| IBIS file 3599z.ibs created by s2ibis2 version 1.1
| North Carolina State University Electronics Research Laboratory  1995
[IBIS ver]   2.1
[File name]   70v3599bf.ibs
[File Rev]   2.0
|1.0 : Original Version - Wei-Ling Chang
|2.0 : Replaced I/O and Input models with 70V659 ADC models - Sunil Kashyap
[Source]   Integrated Device Technology, Inc.
[Notes]   1.Temperatures: typ=25C, min=100C, max=0C 2.RRmp rates based
   on 50 ohm load. 3. Both inpad and iopad have 2 models each.
   (JTAG pins have one model.)
   iopad: standard 3.3V I/O model
   inpad: standard 3.3V input pad model
   iopad25: For 2.5V I/O supply
   inpad25: For 2.5V I/O supply.
   To use 2.%V models at any port, use iopad25 and inpad25
   as the model definition in pin defie section of the IBIS
   file.  JTAG pins only have models for 3.3V I/O voltage.
[Disclaimer] Integrated Device Technology, Inc. ("IDT") hereby grants the
   user of this IBIS model a non-exclusive, nontransferable
   license to use this IBIS model under the following terms. The
   user is granted this license only to use the IBIS model and is
   not granted rights to sell, copy (except as needed to run the
   IBIS model), rent, lease or sub-license the IBIS model in
   whole or in part, or in modified form to anyone. The User may
   modify the IBIS model to suit its specific applications, but
   rights to derivative works and such modifications shall belong
   to IDT. This IBIS model is provided on an AS IS" basis and IDT
   makes absolutely no warranty with respect to the information
   contained herein. IDT DISCLAIMS AND CUSTOMER WAIVES ALL
   WARRANTIES, EXPRESS AND IMPLIED, INCLUDING WARRANTIES OF
   MERCHANTABILITY AND FITNESS FOR A PARTICULAR PURPOSE. THE
   ENTIRE RISK AS TO QUALITY AND PERFORMANCE IS WITH THE USER
   ACCORDINGLY, IN NO EVENT SHALL IDT BE LIABLE FOR ANY DIRECT OR
   INDIRECT DAMAGES, WHETHER IN CONTRACT OR TORT, INCLUDING ANY
   LOST PROFITS OR OTHER INCIDENTAL, CONSEQUENTIAL, EXEMPLARY, OR
   PUNITIVE DAMAGES ARISING OUT OF THE USE OR APPLICATION OF THE
   IBIS model. Further, IDT reserves the right to make changes
   without notice to any product herein to improve reliability,
   function, or design. IDT does not convey any license under
   patent rights or any other intellectual property rights,
   including those of third parties. IDT is not obligated to
   provide maintenance or support for the licensed IBIS model.
[Copyright]   Copyright 2004, Integrated Device Technology, Inc. all rights
   reserved
|   Component idt70v3599z
[Component]   idt70v3599z
[Manufacturer]   Integrated Device Technology
[Package]
| variable   typ   min   max
R_pkg   100.00000m   50.00000m   0.30000
L_pkg   4.00000nH   3.20000nH   5.50000nH
C_pkg   0.64000pF   0.50000pF   0.70000pF
[Pin]  signal_name   model_name   R_pin   L_pin   C_pin
A1   io19l   iopad
C2   io19r   iopad
D4   io20l   iopad
B1   io20r   iopad
C1   VDDQ   POWER
D2   GND   GND
D3   io21l   iopad
E4   io21r   iopad
D1   io22l   iopad
E2   io22r   iopad
E3   VDDQ   POWER
F4   GND   GND
E1   io23l   iopad
F2   io23r   iopad
F3   io24l   iopad
G4   io24r   iopad
F1   VDDQ   POWER
G2   GND   GND
G3   io25l   iopad
H4   io25r   iopad
G1   io26l   iopad
H2   io26r   iopad
H3   VDDQ   POWER
J4   GND   GND
H1   VDD   POWER
J2   VDD   POWER
J3   GND   GND
K4   GND   GND
J1   VDDQ   POWER
K2   GND   GND
K3   io27r   iopad
L4   io27l   iopad
K1   io28r   iopad
L2   io28l   iopad
L3   VDDQ   POWER
M4   GND   GND
L1   io29r   iopad
M2   io29l   iopad
M3   io30r   iopad
N4   io30l   iopad
M1   VDDQ   POWER
N2   GND   GND
N3   io31r   iopad
N1   io31l   iopad
P1   io32r   iopad
P2   io32l   iopad
P3   VDDQ   POWER
R1   GND   GND
T1   io33r   iopad
R2   io33l   iopad
R3   io34r   iopad
T2   io34l   iopad
U1   GND   GND
T3   VDDQ   POWER
P4   io35r   iopad
U2   io35l   iopad
U3   plftr#   inpad
P6   a16r   inpad
U5   a15r   inpad
T6   a14r   inpad
R6   a13r   inpad
P7   a12r   inpad
U6   a11r   inpad
T7   a10r   inpad
R7   a9r   inpad
P8   a8r   inpad
U7   a7r   inpad
T8   be3r#   inpad
R8   be2r#   inpad
P9   be1r#   inpad
U8   be0r#   inpad
T9   ce1r   inpad
R9   ce0r   inpad
P10   VDD   POWER
U9   VDD   POWER
T10   GND   GND
R10   GND   GND
P11   clkr   inpad
U10   oe#   inpad
T11   rwr#   inpad
R11   adsr#   inpad
P12   cntenr#   inpad
U11   repeatr#   inpad
T12   a6r   inpad
R12   a5r   inpad
P13   a4r   inpad
U12   a3r   inpad
T13   a2r   inpad
R13   a1r   inpad
U13   a0r   inpad
U14   VDD   POWER
T14   GND   GND
R14   GND   GND
U15   optr   inpad
U16   io0l   iopad
T15   io0r   iopad
R15   VDDQ   POWER
T16   GND   GND
U17   io1l   iopad
R16   io1r   iopad
P14   io2l   iopad
T17   io2r   iopad
R17   VDDQ   POWER
P16   GND   GND
P15   io3l   iopad
N14   io3r   iopad
P17   io4l   iopad
N16   io4r   iopad
N15   VDDQ   POWER
M14   GND   GND
N17   io5l   iopad
M16   io5r   iopad
M15   io6l   iopad
L14   io6r   iopad
M17   VDDQ   POWER
L16   GND   GND
L15   io7l   iopad
K14   io7r   iopad
L17   io8l   iopad
K16   io8r   iopad
K15   VDDQ   POWER
J14   GND   GND
K17   GND   GND
J16   GND   GND
J15   VDD   POWER
H14   VDD   POWER
J17   VDDQ   POWER
H16   GND   GND
H15   io9r   iopad
G14   io9l   iopad
H17   io10r   iopad
G16   io10l   iopad
G15   VDDQ   POWER
F14   GND   GND
G17   io11r   iopad
F16   io11l   iopad
F15   io12r   iopad
E14   io12l   iopad
F17   VDDQ   POWER
E16   GND   GND
E15   io13r   iopad
E17   io13l   iopad
D17   io14r   iopad
D16   io14l   iopad
D15   VDDQ   POWER
C17   GND   GND
B17   io15r   iopad
C16   io15l   iopad
C15   io16r   iopad
B16   io16l   iopad
A17   GND   GND
B15   VDDQ   POWER
D14   io17r   iopad
A16   io17l   iopad
A15   optl   inpad
B14   GND   GND
C14   VDD   POWER
D13   VDD   POWER
A14   a0l   inpad
B13   a1l   inpad
C13   a2l   inpad
D12   a3l   inpad
A13   a4l   inpad
B12   a5l   inpad
C12   a6l   inpad
A12   cntenl#   inpad
B11   adsl#   inpad
C11   rwl#   inpad
D10   oel#   inpad
A11   clkl   inpad
D11   repeatl#   inpad
B10   GND   GND
C10   GND   GND
D9   VDD   POWER
A10   VDD   POWER
B9   ce0l#   inpad
C9   ce1l   inpad
D8   be0l#   inpad
A9   be1l#   inpad
B8   be2l#   inpad
C8   be3l#   inpad
D7   a7l   inpad
A8   a8l   inpad
B7   a9l   inpad
C7   a10l   inpad
D6   a11l   inpad
A7   a12l   inpad
B6   a13l   inpad
C6   a14l   inpad
D5   a15l   inpad
A6   a16l   inpad
C4   plftl#   inpad
A3   test/GND   GND
A2   io18l   iopad
B3   io18r   iopad
C3   VDDQ   POWER
B2   GND   GND
A4   tdo   iopad
B4   tdi   inpadbs
T4   tms   inpadbs
R4   tck   inpadbs
P5   trst   inpadbs
| in   in   dummy_model
| oe   oe   dummy_model
[Pin Mapping]  pulldown_ref   pullup_ref   gnd_clamp_ref   power_clamp_ref
A1   EXTGND   EXTVDDQ   EXTGND   EXTVDD
C2   EXTGND   EXTVDDQ   EXTGND   EXTVDD
D4   EXTGND   EXTVDDQ   EXTGND   EXTVDD
B1   EXTGND   EXTVDDQ   EXTGND   EXTVDD
C1   NC   EXTVDDQ
D2   EXTGND   NC
D3   EXTGND   EXTVDDQ   EXTGND   EXTVDD
E4   EXTGND   EXTVDDQ   EXTGND   EXTVDD
D1   EXTGND   EXTVDDQ   EXTGND   EXTVDD
E2   EXTGND   EXTVDDQ   EXTGND   EXTVDD
E3   NC   EXTVDDQ
F4   EXTGND   NC
E1   EXTGND   EXTVDDQ   EXTGND   EXTVDD
F2   EXTGND   EXTVDDQ   EXTGND   EXTVDD
F3   EXTGND   EXTVDDQ   EXTGND   EXTVDD
G4   EXTGND   EXTVDDQ   EXTGND   EXTVDD
F1   NC   EXTVDDQ
G2   EXTGND   NC
G3   EXTGND   EXTVDDQ   EXTGND   EXTVDD
H4   EXTGND   EXTVDDQ   EXTGND   EXTVDD
G1   EXTGND   EXTVDDQ   EXTGND   EXTVDD
H2   EXTGND   EXTVDDQ   EXTGND   EXTVDD
H3   NC   EXTVDDQ
J4   EXTGND   NC
H1   NC   EXTVDD
J2   NC   EXTVDD
J3   EXTGND   NC
K4   EXTGND   NC
J1   NC   EXTVDDQ
K2   EXTGND   NC
K3   EXTGND   EXTVDDQ   EXTGND   EXTVDD
L4   EXTGND   EXTVDDQ   EXTGND   EXTVDD
K1   EXTGND   EXTVDDQ   EXTGND   EXTVDD
L2   EXTGND   EXTVDDQ   EXTGND   EXTVDD
L3   NC   EXTVDDQ
M4   EXTGND   NC
L1   EXTGND   EXTVDDQ   EXTGND   EXTVDD
M2   EXTGND   EXTVDDQ   EXTGND   EXTVDD
M3   EXTGND   EXTVDDQ   EXTGND   EXTVDD
N4   EXTGND   EXTVDDQ   EXTGND   EXTVDD
M1   NC   EXTVDDQ
N2   EXTGND   NC
N3   EXTGND   EXTVDDQ   EXTGND   EXTVDD
N1   EXTGND   EXTVDDQ   EXTGND   EXTVDD
P1   EXTGND   EXTVDDQ   EXTGND   EXTVDD
P2   EXTGND   EXTVDDQ   EXTGND   EXTVDD
P3   NC   EXTVDDQ
R1   EXTGND   NC
T1   EXTGND   EXTVDDQ   EXTGND   EXTVDD
R2   EXTGND   EXTVDDQ   EXTGND   EXTVDD
R3   EXTGND   EXTVDDQ   EXTGND   EXTVDD
T2   EXTGND   EXTVDDQ   EXTGND   EXTVDD
U1   EXTGND   NC
T3   NC   EXTVDDQ
P4   EXTGND   EXTVDDQ   EXTGND   EXTVDD
U2   EXTGND   EXTVDDQ   EXTGND   EXTVDD
U3   EXTGND   EXTVDDQ   EXTGND   EXTVDD
P6   EXTGND   EXTVDDQ   EXTGND   EXTVDD
U5   EXTGND   EXTVDDQ   EXTGND   EXTVDD
T6   EXTGND   EXTVDDQ   EXTGND   EXTVDD
R6   EXTGND   EXTVDDQ   EXTGND   EXTVDD
P7   EXTGND   EXTVDDQ   EXTGND   EXTVDD
U6   EXTGND   EXTVDDQ   EXTGND   EXTVDD
T7   EXTGND   EXTVDDQ   EXTGND   EXTVDD
R7   EXTGND   EXTVDDQ   EXTGND   EXTVDD
P8   EXTGND   EXTVDDQ   EXTGND   EXTVDD
U7   EXTGND   EXTVDDQ   EXTGND   EXTVDD
T8   EXTGND   EXTVDDQ   EXTGND   EXTVDD
R8   EXTGND   EXTVDDQ   EXTGND   EXTVDD
P9   EXTGND   EXTVDDQ   EXTGND   EXTVDD
U8   EXTGND   EXTVDDQ   EXTGND   EXTVDD
T9   EXTGND   EXTVDDQ   EXTGND   EXTVDD
R9   EXTGND   EXTVDDQ   EXTGND   EXTVDD
P10   NC   EXTVDD
U9   NC   EXTVDD
T10   EXTGND   NC
R10   EXTGND   NC
P11   EXTGND   EXTVDDQ   EXTGND   EXTVDD
U10   EXTGND   EXTVDDQ   EXTGND   EXTVDD
T11   EXTGND   EXTVDDQ   EXTGND   EXTVDD
R11   EXTGND   EXTVDDQ   EXTGND   EXTVDD
P12   EXTGND   EXTVDDQ   EXTGND   EXTVDD
U11   EXTGND   EXTVDDQ   EXTGND   EXTVDD
T12   EXTGND   EXTVDDQ   EXTGND   EXTVDD
R12   EXTGND   EXTVDDQ   EXTGND   EXTVDD
P13   EXTGND   EXTVDDQ   EXTGND   EXTVDD
U12   EXTGND   EXTVDDQ   EXTGND   EXTVDD
T13   EXTGND   EXTVDDQ   EXTGND   EXTVDD
R13   EXTGND   EXTVDDQ   EXTGND   EXTVDD
U13   EXTGND   EXTVDDQ   EXTGND   EXTVDD
U14   NC   EXTVDD
T14   EXTGND   NC
R14   EXTGND   NC
U15   EXTGND   EXTVDDQ   EXTGND   EXTVDD
U16   EXTGND   EXTVDDQ   EXTGND   EXTVDD
T15   EXTGND   EXTVDDQ   EXTGND   EXTVDD
R15   NC   EXTVDDQ
T16   EXTGND   NC
U17   EXTGND   EXTVDDQ   EXTGND   EXTVDD
R16   EXTGND   EXTVDDQ   EXTGND   EXTVDD
P14   EXTGND   EXTVDDQ   EXTGND   EXTVDD
T17   EXTGND   EXTVDDQ   EXTGND   EXTVDD
R17   NC   EXTVDDQ
P16   EXTGND   NC
P15   EXTGND   EXTVDDQ   EXTGND   EXTVDD
N14   EXTGND   EXTVDDQ   EXTGND   EXTVDD
P17   EXTGND   EXTVDDQ   EXTGND   EXTVDD
N16   EXTGND   EXTVDDQ   EXTGND   EXTVDD
N15   NC   EXTVDDQ
M14   EXTGND   NC
N17   EXTGND   EXTVDDQ   EXTGND   EXTVDD
M16   EXTGND   EXTVDDQ   EXTGND   EXTVDD
M15   EXTGND   EXTVDDQ   EXTGND   EXTVDD
L14   EXTGND   EXTVDDQ   EXTGND   EXTVDD
M17   NC   EXTVDDQ
L16   EXTGND   NC
L15   EXTGND   EXTVDDQ   EXTGND   EXTVDD
K14   EXTGND   EXTVDDQ   EXTGND   EXTVDD
L17   EXTGND   EXTVDDQ   EXTGND   EXTVDD
K16   EXTGND   EXTVDDQ   EXTGND   EXTVDD
K15   NC   EXTVDDQ
J14   EXTGND   NC
K17   EXTGND   NC
J16   EXTGND   NC
J15   NC   EXTVDD
H14   NC   EXTVDD
J17   NC   EXTVDDQ
H16   EXTGND   NC
H15   EXTGND   EXTVDDQ   EXTGND   EXTVDD
G14   EXTGND   EXTVDDQ   EXTGND   EXTVDD
H17   EXTGND   EXTVDDQ   EXTGND   EXTVDD
G16   EXTGND   EXTVDDQ   EXTGND   EXTVDD
G15   NC   EXTVDDQ
F14   EXTGND   NC
G17   EXTGND   EXTVDDQ   EXTGND   EXTVDD
F16   EXTGND   EXTVDDQ   EXTGND   EXTVDD
F15   EXTGND   EXTVDDQ   EXTGND   EXTVDD
E14   EXTGND   EXTVDDQ   EXTGND   EXTVDD
F17   NC   EXTVDDQ
E16   EXTGND   NC
E15   EXTGND   EXTVDDQ   EXTGND   EXTVDD
E17   EXTGND   EXTVDDQ   EXTGND   EXTVDD
D17   EXTGND   EXTVDDQ   EXTGND   EXTVDD
D16   EXTGND   EXTVDDQ   EXTGND   EXTVDD
D15   NC   EXTVDDQ
C17   EXTGND   NC
B17   EXTGND   EXTVDDQ   EXTGND   EXTVDD
C16   EXTGND   EXTVDDQ   EXTGND   EXTVDD
C15   EXTGND   EXTVDDQ   EXTGND   EXTVDD
B16   EXTGND   EXTVDDQ   EXTGND   EXTVDD
A17   EXTGND   NC
B15   NC   EXTVDDQ
D14   EXTGND   EXTVDDQ   EXTGND   EXTVDD
A16   EXTGND   EXTVDDQ   EXTGND   EXTVDD
A15   EXTGND   EXTVDDQ   EXTGND   EXTVDD
B14   EXTGND   NC
C14   NC   EXTVDD
D13   NC   EXTVDD
A14   EXTGND   EXTVDDQ   EXTGND   EXTVDD
B13   EXTGND   EXTVDDQ   EXTGND   EXTVDD
C13   EXTGND   EXTVDDQ   EXTGND   EXTVDD
D12   EXTGND   EXTVDDQ   EXTGND   EXTVDD
A13   EXTGND   EXTVDDQ   EXTGND   EXTVDD
B12   EXTGND   EXTVDDQ   EXTGND   EXTVDD
C12   EXTGND   EXTVDDQ   EXTGND   EXTVDD
A12   EXTGND   EXTVDDQ   EXTGND   EXTVDD
B11   EXTGND   EXTVDDQ   EXTGND   EXTVDD
C11   EXTGND   EXTVDDQ   EXTGND   EXTVDD
D10   EXTGND   EXTVDDQ   EXTGND   EXTVDD
A11   EXTGND   EXTVDDQ   EXTGND   EXTVDD
D11   EXTGND   EXTVDDQ   EXTGND   EXTVDD
B10   EXTGND   NC
C10   EXTGND   NC
D9   NC   EXTVDD
A10   NC   EXTVDD
B9   EXTGND   EXTVDDQ   EXTGND   EXTVDD
C9   EXTGND   EXTVDDQ   EXTGND   EXTVDD
D8   EXTGND   EXTVDDQ   EXTGND   EXTVDD
A9   EXTGND   EXTVDDQ   EXTGND   EXTVDD
B8   EXTGND   EXTVDDQ   EXTGND   EXTVDD
C8   EXTGND   EXTVDDQ   EXTGND   EXTVDD
D7   EXTGND   EXTVDDQ   EXTGND   EXTVDD
A8   EXTGND   EXTVDDQ   EXTGND   EXTVDD
B7   EXTGND   EXTVDDQ   EXTGND   EXTVDD
C7   EXTGND   EXTVDDQ   EXTGND   EXTVDD
D6   EXTGND   EXTVDDQ   EXTGND   EXTVDD
A7   EXTGND   EXTVDDQ   EXTGND   EXTVDD
B6   EXTGND   EXTVDDQ   EXTGND   EXTVDD
C6   EXTGND   EXTVDDQ   EXTGND   EXTVDD
D5   EXTGND   EXTVDDQ   EXTGND   EXTVDD
A6   EXTGND   EXTVDDQ   EXTGND   EXTVDD
C4   EXTGND   EXTVDDQ   EXTGND   EXTVDD
A3   EXTGND   NC
A2   EXTGND   EXTVDDQ   EXTGND   EXTVDD
B3   EXTGND   EXTVDDQ   EXTGND   EXTVDD
C3   NC   EXTVDDQ
B2   EXTGND   NC
A4   EXTGND   EXTVDDQ   EXTGND   EXTVDD
B4   EXTGND   EXTVDDQ   EXTGND   EXTVDD
T4   EXTGND   EXTVDDQ   EXTGND   EXTVDD
R4   EXTGND   EXTVDDQ   EXTGND   EXTVDD
P5   EXTGND   EXTVDDQ   EXTGND   EXTVDD
| Models and submodels in the file (5): iopad (I/O), inpad (Input), inpadbs (Input), iopad25 (I/O), inpad25 (Input)
